FUNCTION_BLOCK FB_DataFifo
VAR_INPUT
	bPutData	:	BOOL;
	bGetData	:	BOOL;
	bClearFifo	:	BOOL;
	pPutData	:	pvoid;
	pGetData	:	pvoid;
	nDataLen	:	UDINT;
	pFifoMemory	:	pvoid;
	nFifoSize	:	DINT;

END_VAR
VAR_OUTPUT
	bFifoEmpty	:	BOOL;
	bFifoFull	:	BOOL;
	iFifoSizeLeft	: DINT;
END_VAR
VAR
	fbGetTaskId	: GETCURTASKINDEX;
	nTaskId		: BYTE;
	
	iPutIndex	:	DINT;
	iGetIndex	:	DINT;

	pPutIndex	:	DINT;
	pGetIndex	:	DINT;
	bIs1Sec : BOOL;

END_VAR


IF bClearFifo THEN
	iPutIndex := 0; iGetIndex := 0;
	iFifoSizeLeft := nFifoSize;
	bFifoEmpty := TRUE;
	RETURN;
END_IF

IF NOT(bFifoFull) THEN
	IF bPutData THEN
		IF iPutIndex >= nFifoSize THEN
			iPutIndex := 0;
		END_IF
		pPutIndex := iPutIndex * nDataLen;
		MEMCPY(pFifoMemory + pPutIndex, pPutData, nDataLen);
		iPutIndex := iPutIndex + 1;
		iFifoSizeLeft := iFifoSizeLeft - 1;
	END_IF
END_IF;

IF NOT(bFifoEmpty) THEN
	IF bGetData THEN
		bIs1Sec := iGetIndex >= nFifoSize;
		
		IF bIs1Sec THEN
			iGetIndex := 0;
		END_IF
		pGetIndex := iGetIndex * nDataLen;
		MEMCPY(pGetData, pFifoMemory + pGetIndex , nDataLen);
		iGetIndex := iGetIndex + 1;
		iFifoSizeLeft := iFifoSizeLeft + 1;
	END_IF
END_IF;


(*
 _TaskInfo[GETCURTASKINDEX()].FirstCycle;
SystemTaskInfoArr[SystemInfo.RuntimeNo].firstCycle
*)


fbGetTaskId();	
IF _TaskInfo[fbGetTaskId.index].FirstCycle THEN
	iFifoSizeLeft  := nFifoSize;
END_IF

//IF iFifoSizeLeft = 0 THEN
//	bFifoFull := TRUE;
//ELSE
//	bFifoFull := FALSE;
//END_IF

//IF iFifoSizeLeft >= nFifoSize THEN
//	bFifoEmpty := TRUE;
//ELSE
//	bFifoEmpty := FALSE;
//END_IF

END_FUNCTION_BLOCK
